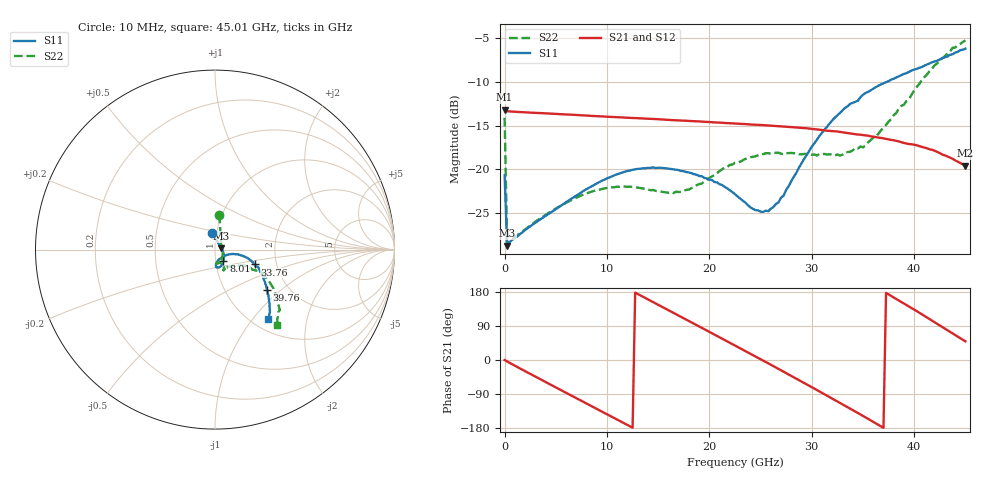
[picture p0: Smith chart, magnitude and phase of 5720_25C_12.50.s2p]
! Device:  ADRF5720
! Description: 0.5dB LSB GaAs MMIC 6-bit Digital Attenuator
! Frequency:  0.000009 -  40 GHz
! Ports:
!	RF1	= Port 1
!	RF2	= Port 2
! Vdd:  3.3 Volt
! Vss:  -3.3 Volt
! Control:  0/3.3 Volt
! State:  12.50 dB attenuation
! Data:  The device was measured using G-S-G Probes on a matrix board.
!  Data was collected using an calibrated 4 port network analyzer.
!  The reference plane for this measurement is at the launchers.
! Note:  Analog Devices supplies this data as a sample of measured data
!  for this product.  Your particular data for this product may vary.
!  Data was taken at 25 degrees C.
!  Analog Devices reserves the right to change this data at anytime.
# GHZ S DB R 45.0
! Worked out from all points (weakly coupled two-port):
!   181 points, 10 MHz to 45.01 GHz, reference 45 ohm
!   highest |S21| = -13.18 dB at 10 MHz (marker M1); lowest = -19.6 dB at 45.01 GHz (marker M2)
!   lowest |S11| = -28.7 dB at 260 MHz (marker M3), VSWR 1.08, Z = 48.3 + j0.785 ohm
!   |S11| at or under -10 dB: start of sweep to 37.35 GHz
!   |S22| runs from -28.8 to -5.3 dB; largest |S21 - S12| = 0.00032
!   S11 on the Smith chart (normalised r, x): 10 MHz: 0.95, +0.18; 8.01 GHz: 1.09, -0.13; 33.76 GHz: 1.54, -0.27; 39.76 GHz: 1.56, -0.81; 45.01 GHz: 1.18, -1.20
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0.01  -20.66 99.9  -13.18 -0.1  -13.18 -0.1  -14.11 82.9
0.26  -28.72 12.8  -13.37 -4.0  -13.38 -4.0  -28.78 11.4
2.01  -26.95 -10.2  -13.49 -29.5  -13.49 -29.5  -26.86 -18.2
4.26  -25.12 -29.9  -13.62 -61.6  -13.63 -61.6  -25.02 -43.3
7.76  -22.43 -50.9  -13.84 -111.4  -13.84 -111.3  -22.86 -67.3
8.01  -22.26 -52.3  -13.86 -114.9  -13.86 -114.9  -22.74 -68.6
11.76  -20.28 -69.6  -14.09 -168.0  -14.10 -168.0  -21.97 -82.1
15.26  -19.82 -81.4  -14.29 142.1  -14.30 142.1  -22.55 -82.4
17.26  -20.19 -85.3  -14.43 113.6  -14.43 113.6  -22.55 -74.5
19.01  -20.77 -86.8  -14.53 88.5  -14.54 88.6  -21.69 -66.8
22.76  -23.10 -81.0  -14.79 34.7  -14.79 34.7  -19.23 -63.2
24.26  -24.53 -68.7  -14.90 13.0  -14.90 13.1  -18.57 -64.7
25.76  -24.79 -46.3  -14.99 -8.8  -14.99 -8.8  -18.16 -66.4
27.26  -23.01 -24.8  -15.10 -30.9  -15.11 -30.9  -18.28 -66.7
30.26  -17.01 -11.9  -15.41 -75.5  -15.42 -75.4  -18.31 -63.6
33.76  -12.52 -20.5  -15.90 -128.4  -15.90 -128.4  -17.99 -48.1
35.26  -11.28 -24.4  -16.12 -151.5  -16.12 -151.5  -17.28 -40.2
37.76  -9.75 -32.3  -16.64 169.2  -16.64 169.3  -14.28 -27.8
39.76  -8.72 -37.9  -17.14 137.3  -17.14 137.4  -11.46 -26.5
42.01  -7.69 -43.2  -17.88 99.3  -17.88 99.4  -8.11 -33.7
43.76  -6.85 -48.0  -18.80 69.9  -18.79 70.0  -6.12 -43.0
45.01  -6.22 -52.5  -19.60 49.3  -19.60 49.4  -5.28 -50.3
